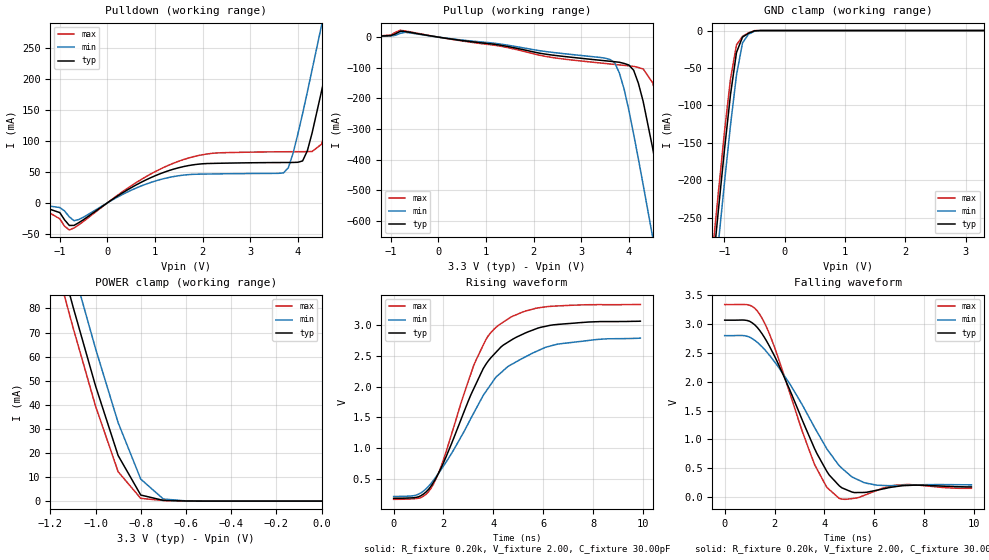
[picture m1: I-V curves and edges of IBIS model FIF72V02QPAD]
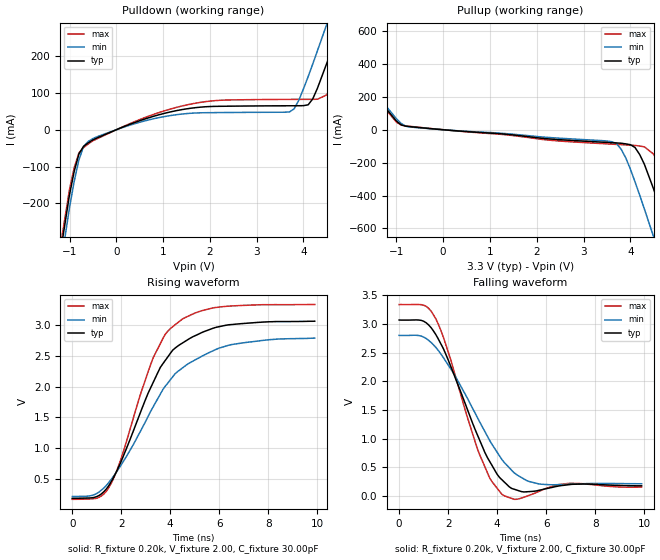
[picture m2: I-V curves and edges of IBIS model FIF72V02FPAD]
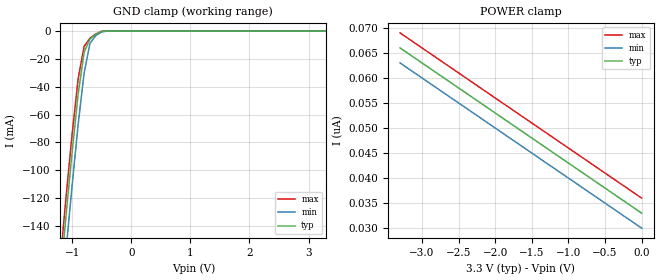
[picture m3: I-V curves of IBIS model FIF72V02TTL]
| IBIS file i72v82.ibs created by s2ibis2 version 1.1
| North Carolina State University Electronics Research Laboratory  1995
[IBIS ver]   2.1
[File name]   i72v82.ibs
[File Rev]   1.0
[Date]   07/22/98
[Source]   Integrated Device Technology, Inc.
[Notes]   1. Temperatures: typ=25C, min=70C, max=0C 2. Cemos8_5v
   process. 3. Ramp rates based on 50 ohm load.
[Copyright]   Copyright 1997, Integrated Device Technology, Inc.
|   Component idt72V82
[Component]   idt72V82
[Manufacturer]   Integrated Device Technology
[Package]
| variable   typ   min   max
R_pkg   0.75   0.60   0.90
L_pkg   8.10nH   8.30nH   9.90nH
C_pkg   0.53pF   0.46pF   0.60pF
[Pin]  signal_name   model_name   R_pin   L_pin   C_pin
1   FFAL   FIF72V02FPAD
2   QA0   FIF72V02QPAD
3   QA1   FIF72V02QPAD
4   QA2   FIF72V02QPAD
5   QA3   FIF72V02QPAD
6   QA8   FIF72V02QPAD
7   GND   GND
8   RAL   FIF72V02TTL
9   QA4   FIF72V02QPAD
10   QA5   FIF72V02QPAD
11   QA6   FIF72V02QPAD
12   QA7   FIF72V02QPAD
13   XOLHFAL   FIF72V02FPAD
14   EFAL   FIF72V02FPAD
15   FFBL   FIF72V02FPAD
16   QB0   FIF72V02QPAD
17   QB1   FIF72V02QPAD
18   QB2   FIF72V02QPAD
19   QB3   FIF72V02QPAD
20   QB8   FIF72V02QPAD
21   GND   GND
22   RBL   FIF72V02TTL
23   QB4   FIF72V02QPAD
24   QB5   FIF72V02QPAD
25   QB6   FIF72V02QPAD
26   QB7   FIF72V02QPAD
27   XOLHFBL   FIF72V02FPAD
28   EFBL   FIF72V02FPAD
29   RSBL   FIF72V02TTL
30   FLRTBL   FIF72V02TTL
31   DB7   FIF72V02TTL
32   DB6   FIF72V02TTL
33   DB5   FIF72V02TTL
34   DB4   FIF72V02TTL
35   VCC   POWER
36   WBL   FIF72V02TTL
37   DB8   FIF72V02TTL
38   DB3   FIF72V02TTL
39   DB2   FIF72V02TTL
40   DB1   FIF72V02TTL
41   DB0   FIF72V02TTL
42   XIBL   FIF72V02TTL
43   RSAL   FIF72V02TTL
44   FLRTAL   FIF72V02TTL
45   DA7   FIF72V02TTL
46   DA6   FIF72V02TTL
47   DA5   FIF72V02TTL
48   DA4   FIF72V02TTL
49   VCC   POWER
50   WAL   FIF72V02TTL
51   DA8   FIF72V02TTL
52   DA3   FIF72V02TTL
53   DA2   FIF72V02TTL
54   DA1   FIF72V02TTL
55   DA0   FIF72V02TTL
56   XIAL   FIF72V02TTL
| Models and submodels in the file (3): FIF72V02QPAD (3-state), FIF72V02FPAD (Output), FIF72V02TTL (Input)
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| FIN  FIN   dummy_model
| QIN  QIN   dummy_model
| QOEL QOEL   dummy_model
|   Model FIF72V02QPAD
[Model]   FIF72V02QPAD
Model_type   3-state
Polarity   Non-Inverting
Enable   Active-Low
Vmeas =  1.500V
C_comp   3.00pF   NA   NA
[Temperature Range]   25.00   70.00   0.000
[Voltage Range]   3.30V   3.00V   3.60V
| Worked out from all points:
|   slope of the pulldown table from 0 to 0.495 V, typ, clamps not added: 20.4 ohm
|   slope of the pullup table from 0 to 0.495 V, typ, clamps not added: 44.7 ohm
|   GND clamp passes 1 mA (typ) near -0.52 V on its own axis
|   POWER clamp passes 1 mA (typ) near -0.73 V on its own axis
|   rising waveform, R_fixture 0.20k, V_fixture 2.00, C_fixture 30.00pF: 20-80 % time 1.95ns typ, 2.41ns min, 1.64ns max; typ from 0.181 V to 3.07 V
|   falling waveform, R_fixture 0.20k, V_fixture 2.00, C_fixture 30.00pF: 20-80 % time 1.76ns typ, 2.17ns min, 1.5ns max; typ from 3.07 V to 0.177 V
[Pulldown]
| voltage   I(typ)   I(min)   I(max)
-3.3V     -1mA       -1mA       0A
-1.5V     -2.7mA     -2.1mA     -3.3mA
-800mV    -36.55mA   -22.69mA   -43.77mA
1.5V      56.64mA    43.75mA    67.16mA
3.7V      65mA       48.37mA    82.35mA
3.9V      65.11mA    80.12mA    82.43mA
4.1V      67.6mA     144mA      82.48mA
4.5V      181mA      287mA      94.75mA
4.7V      253mA      361mA      155mA
4.9V      326mA      435mA      225mA
5.1V      400mA      510mA      298mA
6.6V      966mA      1.076A     862mA
[Pullup]
| voltage   I(typ)   I(min)   I(max)
-3.3V     300uA      300uA      300uA
-800mV    19.13mA    12.44mA    22.38mA
3.6V      -78.68mA   -72.88mA   -87.52mA
3.7V      -80.24mA   -82.94mA   -89.09mA
3.9V      -85.87mA   -170mA     -92.22mA
4.1V      -108mA     -317mA     -95.4mA
4.3V      -210mA     -482mA     -104mA
4.5V      -363mA     -653mA     -149mA
4.7V      -531mA     -826mA     -270mA
4.9V      -703mA     -1A        -430mA
5.1V      -878mA     -1.176A    -601mA
6.6V      -2.207A    -2.508A    -1.926A
[GND_clamp]
| voltage   I(typ)   I(min)   I(max)
-3.3V     -2.171A    -2.212A    -2.149A
-1.2V     -323mA     -367mA     -298mA
-1.1V     -240mA     -284mA     -216mA
-1V       -160mA     -204mA     -136mA
-900mV    -86.07mA   -127mA     -65.05mA
-800mV    -29.34mA   -59.59mA   -19.24mA
-700mV    -8.788mA   -16.49mA   -7.804mA
-600mV    -3.672mA   -4.887mA   -3.17mA
-500mV    -365uA     -944uA     -138uA
-400mV    -14.29nA   -611nA     -4.611nA
3.3V      33nA       33.88nA    33nA
[POWER_clamp]
| voltage   I(typ)   I(min)   I(max)
-3.3V     901mA      915mA      893mA
-1.2V     116mA      132mA      107mA
-1.1V     80.92mA    96.84mA    72.29mA
-1V       47.89mA    63.39mA    39.51mA
-900mV    18.95mA    32.6mA     12.21mA
-800mV    2.533mA    9.147mA    1.14mA
-700mV    314uA      878uA      268uA
-600mV    64.82uA    96.03uA    58.5uA
0V        33nA       30nA       36nA
[Ramp]
| variable   typ   min   max
dV/dt_r   1.03/1.09n   0.87/1.27n   1.19/0.99n
dV/dt_f   1.35/1.45n   1.13/1.85n   1.54/1.17n
R_load = 50.00
[Rising Waveform]
R_fixture = 0.20k
V_fixture = 2.00
C_fixture = 30.00pF
R_dut = 0.75
L_dut = 8.10nH
C_dut = 0.53pF
| time   V(typ)   V(min)   V(max)
0s        181mV      211mV      165mV
1ns       207mV      250mV      183mV
1.5ns     380mV      424mV      346mV
2ns       761mV      708mV      812mV
3.2ns     1.956V     1.561V     2.333V
3.7ns     2.364V     1.92V      2.767V
4.2ns     2.601V     2.19V      2.998V
5.2ns     2.859V     2.468V     3.22V
6.4ns     3.007V     2.675V     3.312V
9.9ns     3.067V     2.791V     3.339V
[Falling Waveform]
R_fixture = 0.20k
V_fixture = 2.00
C_fixture = 30.00pF
R_dut = 0.75
L_dut = 8.10nH
C_dut = 0.53pF
| time   V(typ)   V(min)   V(max)
0s        3.068V     2.8V       3.338V
1ns       3.048V     2.773V     3.327V
1.5ns     2.831V     2.606V     3.1V
2ns       2.445V     2.345V     2.598V
3.6ns     846mV      1.212V     571mV
4.1ns     445mV      835mV      168mV
4.6ns     195mV      542mV      -23.03mV
6.1ns     119mV      207mV      115mV
7.3ns     201mV      207mV      218mV
9.9ns     177mV      213mV      152mV
|   Model FIF72V02FPAD
[Model]   FIF72V02FPAD
Model_type   Output
Vmeas =  1.500V
C_comp   3.00pF   NA   NA
[Temperature Range]   25.00   70.00   0.000
[Voltage Range]   3.30V   3.00V   3.60V
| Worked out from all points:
|   slope of the pulldown table from 0 to 0.495 V, typ, clamps not added: 20.4 ohm
|   slope of the pullup table from 0 to 0.495 V, typ, clamps not added: 44.7 ohm
|   rising waveform, R_fixture 0.20k, V_fixture 2.00, C_fixture 30.00pF: 20-80 % time 1.94ns typ, 2.4ns min, 1.63ns max; typ from 0.181 V to 3.07 V
|   falling waveform, R_fixture 0.20k, V_fixture 2.00, C_fixture 30.00pF: 20-80 % time 1.62ns typ, 2.05ns min, 1.36ns max; typ from 3.07 V to 0.176 V
[Pulldown]
| voltage   I(typ)   I(min)   I(max)
-3.3V     2.793A     -2.213A    -2.149A
-3.1V     -1.993A    -2.035A    -1.971A
-1.5V     -582mA     -626mA     -558mA
-1V       -176mA     -211mA     -162mA
-800mV    -65.89mA   -82.28mA   -63.01mA
-400mV    -21.63mA   -18.48mA   -23.86mA
1.6V      58.46mA    44.74mA    69.8mA
3.7V      65mA       48.37mA    82.35mA
4.1V      67.6mA     144mA      82.48mA
4.5V      181mA      287mA      94.75mA
5.1V      400mA      510mA      298mA
6.6V      966mA      1.076A     862mA
[Pullup]
| voltage   I(typ)   I(min)   I(max)
-3.3V     901mA      915mA      893mA
-2.5V     598mA      613mA      590mA
-900mV    29.8mA     38.77mA    28.31mA
3.6V      -78.68mA   -72.88mA   -87.52mA
3.9V      -85.87mA   -170mA     -92.22mA
4.1V      -108mA     -317mA     -95.4mA
4.3V      -210mA     -482mA     -104mA
4.5V      -363mA     -653mA     -149mA
4.7V      -531mA     -826mA     -270mA
4.9V      -703mA     -1A        -430mA
5.1V      -878mA     -1.176A    -601mA
6.6V      -2.207A    -2.508A    -1.926A
[Ramp]
| variable   typ   min   max
dV/dt_r   1.03/1.07n   0.87/1.29n   1.19/0.96n
dV/dt_f   1.35/1.23n   1.13/1.60n   1.54/1.03n
R_load = 50.00
[Rising Waveform]
R_fixture = 0.20k
V_fixture = 2.00
C_fixture = 30.00pF
R_dut = 0.75
L_dut = 8.10nH
C_dut = 0.53pF
| time   V(typ)   V(min)   V(max)
0s        181mV      211mV      165mV
1ns       210mV      260mV      183mV
1.5ns     393mV      443mV      363mV
2ns       788mV      728mV      837mV
3.3ns     2.067V     1.67V      2.468V
3.8ns     2.43V      2.009V     2.856V
4.1ns     2.595V     2.161V     2.978V
5.1ns     2.846V     2.454V     3.213V
6.4ns     3.009V     2.676V     3.312V
9.9ns     3.067V     2.791V     3.339V
[Falling Waveform]
R_fixture = 0.20k
V_fixture = 2.00
C_fixture = 30.00pF
R_dut = 0.75
L_dut = 8.10nH
C_dut = 0.53pF
| time   V(typ)   V(min)   V(max)
0s        3.068V     2.8V       3.338V
1ns       3.047V     2.771V     3.327V
1.5ns     2.812V     2.59V      3.088V
3.2ns     1.059V     1.362V     814mV
3.7ns     598mV      964mV      309mV
4.2ns     280mV      631mV      25.41mV
5ns       74.15mV    319mV      -37.61mV
5.7ns     96.8mV     209mV      77.59mV
7ns       200mV      204mV      221mV
9.9ns     176mV      212mV      154mV
|   Model FIF72V02TTL
[Model]   FIF72V02TTL
Model_type   Input
Vinl =  0.000V
Vinh =  3.000V
Vmeas =  1.500V
C_comp   3.00pF   NA   NA
[Temperature Range]   25.00   70.00   0.000
[Voltage Range]   3.30V   3.00V   3.60V
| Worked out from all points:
|   GND clamp passes 1 mA (typ) near -0.54 V on its own axis
[GND_clamp]
| voltage   I(typ)   I(min)   I(max)
-3.3V     -1.215A    -1.238A    -1.203A
-1.2V     -177mA     -201mA     -164mA
-1.1V     -130mA     -155mA     -117mA
-1V       -85.9mA    -110mA     -73.09mA
-900mV    -45.15mA   -67.03mA   -34.14mA
-800mV    -15.42mA   -30.38mA   -11.05mA
-700mV    -5.554mA   -8.773mA   -5.066mA
-600mV    -2.384mA   -3.102mA   -2.034mA
-500mV    -209uA     -595uA     -61.81uA
-400mV    -8.386nA   -263nA     -4.26nA
3.3V      33nA       33nA       33nA
[POWER_clamp]
| voltage   I(typ)   I(min)   I(max)
-3.3V     66nA       63nA       69nA
-3.2V     65nA       62nA       68nA
-3V       63nA       60nA       66nA
0V        33nA       30nA       36nA
